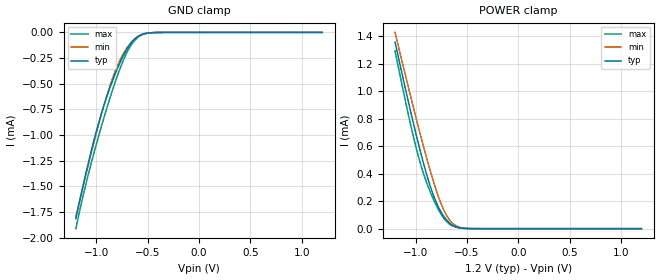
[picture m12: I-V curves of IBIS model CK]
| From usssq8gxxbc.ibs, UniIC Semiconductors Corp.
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|   Model CK
[Model] CK
Model_type Input
Polarity   Non-Inverting
Enable   Active-High
Vinl =  5.100E-01
Vinh =  6.900E-01
C_comp   3.480E-13   3.325E-13   3.631E-13
C_comp_power_clamp   1.016E-13   9.478E-14   1.066E-13
C_comp_gnd_clamp   6.227E-14   6.141E-14   6.489E-14
[Model Spec]
Vinh   6.900E-01   6.600E-01   7.200E-01
Vinl   5.100E-01   4.800E-01   5.400E-01
[Temperature Range]   4.500E+01   9.500E+01   0.000E+00
[Voltage Range]   1.200E+00   1.140E+00   1.260E+00
[C Comp Corner]
C_comp_power_clamp   1.016E-13   9.478E-14   1.066E-13
C_comp_gnd_clamp   6.227E-14   6.141E-14   6.489E-14
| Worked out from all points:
|   GND clamp passes 1 mA (typ) near -1.01 V on its own axis
|   POWER clamp passes 1 mA (typ) near -1.09 V on its own axis
[GND_clamp]
|Voltage   I(typ)   I(min)   I(max)
-1.2V     -1.816mA   -1.797mA   -1.913mA
-1.125V   -1.474mA   -1.481mA   -1.574mA
-1.025V   -1.057mA   -1.076mA   -1.18mA
-950mV    -787.4uA   -793.9uA   -912.4uA
-850mV    -490.5uA   -468.5uA   -584.5uA
-800mV    -364.5uA   -337.8uA   -436uA
-725mV    -204.3uA   -187.1uA   -243.5uA
-675mV    -121.3uA   -114.6uA   -144.9uA
-600mV    -42.01uA   -44.1uA    -50.98uA
-525mV    -10.75uA   -12.45uA   -11.9uA
-425mV    -1.264uA   -1.773uA   -1.033uA
1.2V      0A         0A         0A
[POWER_clamp]
|Voltage   I(typ)   I(min)   I(max)
-1.2V     1.357mA    1.427mA    1.293mA
-1.1V     1.021mA    1.119mA    932.1uA
-1.025V   779.4uA    893uA      681.4uA
-975mV    625.7uA    746.2uA    532.4uA
-925mV    481.4uA    603.8uA    405.6uA
-850mV    293uA      402.8uA    254.4uA
-775mV    153.6uA    227.5uA    135.3uA
-700mV    64.9uA     98.55uA    53.69uA
-625mV    19.09uA    30.19uA    15.19uA
-550mV    3.884uA    6.337uA    3.056uA
-450mV    301.8nA    547.4nA    205.5nA
1.2V      0A         0A         0A
